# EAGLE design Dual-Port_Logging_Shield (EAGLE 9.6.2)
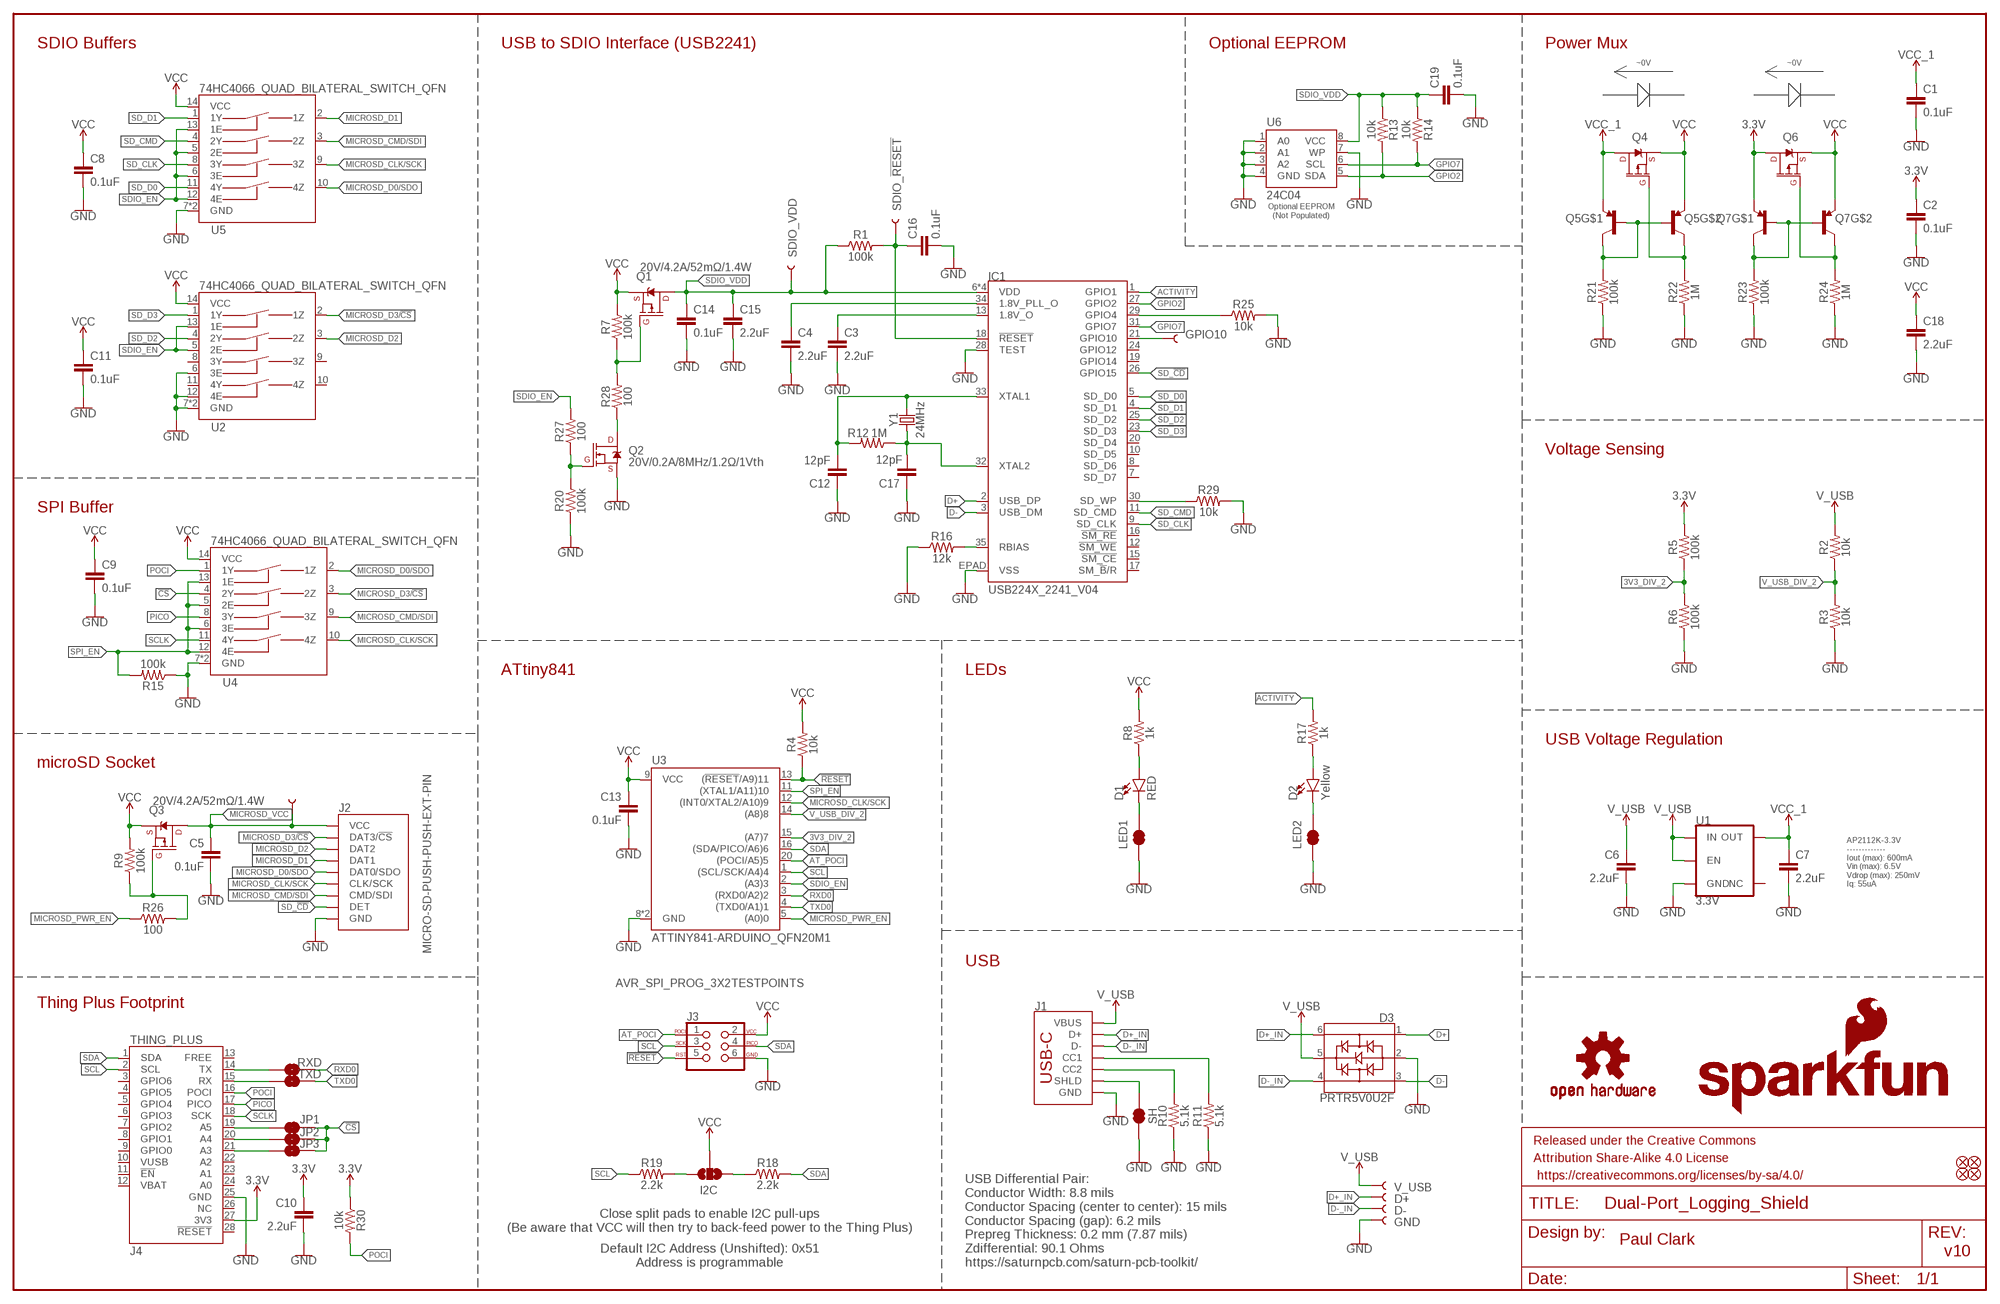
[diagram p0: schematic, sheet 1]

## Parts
C1  0.1uF  0.1UF-0402T-6.3V-10%-X7R  [0402-TIGHT]
C2  0.1uF  0.1UF-0402T-6.3V-10%-X7R  [0402-TIGHT]
C3  2.2uF  2.2UF-0402_TIGHT-10V-10%-X5R  [0402-TIGHT]
C4  2.2uF  2.2UF-0402_TIGHT-10V-10%-X5R  [0402-TIGHT]
C5  0.1uF  0.1UF-0402T-6.3V-10%-X7R  [0402-TIGHT]
C6  2.2uF  2.2UF-0402_TIGHT-10V-10%-X5R  [0402-TIGHT]
C7  2.2uF  2.2UF-0402_TIGHT-10V-10%-X5R  [0402-TIGHT]
C8  0.1uF  0.1UF-0402T-6.3V-10%-X7R  [0402-TIGHT]
C9  0.1uF  0.1UF-0402T-6.3V-10%-X7R  [0402-TIGHT]
C10  2.2uF  2.2UF-0402_TIGHT-10V-10%-X5R  [0402-TIGHT]
C11  0.1uF  0.1UF-0402T-6.3V-10%-X7R  [0402-TIGHT]
C12  12pF  12PF-0402T-50V-5%  [0402-TIGHT]
C13  0.1uF  0.1UF-0402T-6.3V-10%-X7R  [0402-TIGHT]
C14  0.1uF  0.1UF-0402T-6.3V-10%-X7R  [0402-TIGHT]
C15  2.2uF  2.2UF-0402_TIGHT-10V-10%-X5R  [0402-TIGHT]
C16  0.1uF  0.1UF-0402T-6.3V-10%-X7R  [0402-TIGHT]
C17  12pF  12PF-0402T-50V-5%  [0402-TIGHT]
C18  2.2uF  2.2UF-0402_TIGHT-10V-10%-X5R  [0402-TIGHT]
C19  0.1uF  0.1UF-0402T-6.3V-10%-X7R  [0402-TIGHT]
D1  RED  LED-RED0603  [LED-0603]
D2  Yellow  LED-YELLOW0603  [LED-0603]
D3  PRTR5V0U2F  [SOT886]
D+  TEST-POINT3X5  [PAD.03X.05]
D-  TEST-POINT3X5  [PAD.03X.05]
FD1  FIDUCIALUFIDUCIAL  [FIDUCIAL-MICRO]
FD2  FIDUCIALUFIDUCIAL  [FIDUCIAL-MICRO]
FD3  FIDUCIALUFIDUCIAL  [FIDUCIAL-MICRO]
FD4  FIDUCIALUFIDUCIAL  [FIDUCIAL-MICRO]
FRAME1  FRAME-LEDGER  [CREATIVE_COMMONS]
GND  TEST-POINT3X5  [PAD.03X.05]
GPIO10  TEST-POINT3  [PAD.03X.03]
I2C  JUMPER-SMT_3_NO_SILK  [SMT-JUMPER_3_NO_SILK]
IC1  USB224X_2241_V04  [36-QFN]
J1  USB_C_4-LAYER_PADS  [USB-C-16P_4LAYER-PADS]
J2  MICRO-SD-PUSH-PUSH-EXT-PIN  [MICROSD-EXTERNALPIN]
J3  AVR_SPI_PROG_3X2TESTPOINTS  [2X3_TEST_POINTS]
J4  THING_PLUS  [THING_PLUS]
JP1  JUMPER-SMT_2_NC_TRACE_SILK  [SMT-JUMPER_2_NC_TRACE_SILK]
JP2  JUMPER-SMT_2_NO_SILK  [SMT-JUMPER_2_NO_SILK]
JP3  JUMPER-SMT_2_NO_SILK  [SMT-JUMPER_2_NO_SILK]
LED1  JUMPER-SMT_2_NC_TRACE_SILK  [SMT-JUMPER_2_NC_TRACE_SILK]
LED2  JUMPER-SMT_2_NC_TRACE_SILK  [SMT-JUMPER_2_NC_TRACE_SILK]
LOGO2  OSHW-LOGOMINI  [OSHW-LOGO-MINI]
LOGO3  OSHW-LOGOMINI  [OSHW-LOGO-MINI]
LOGO4  SFE_LOGO_FLAME.2_INCH  [SFE_LOGO_FLAME_.2]
LOGO5  SFE_LOGO_NAME_FLAME.1_INCH  [SFE_LOGO_NAME_FLAME_.1]
MICROSD_VCC  TEST-POINT3  [PAD.03X.03]
Q1  20V/4.2A/52mΩ/1.4W  MOSFET_PCH-DMG2305UX-7  [SOT23-3]
Q2  20V/0.2A/8MHz/1.2Ω/1Vth  MOSFET-NCH-RE1C002UNTCL  [SOT-416FL]
Q3  20V/4.2A/52mΩ/1.4W  MOSFET_PCH-DMG2305UX-7  [SOT23-3]
Q4  20V/4.2A/52mΩ/1.4W  MOSFET_PCH-DMG2305UX-7  [SOT23-3]
Q5  TRANS_PNP_DUALSOT-363  [SOT363_PHILIPS]
Q6  20V/4.2A/52mΩ/1.4W  MOSFET_PCH-DMG2305UX-7  [SOT23-3]
Q7  TRANS_PNP_DUALSOT-363  [SOT363_PHILIPS]
R1  100k  100KOHM-0402T-1/16W-1%  [0402-TIGHT]
R2  10k  10KOHM-0402T-1/16W-1%  [0402-TIGHT]
R3  10k  10KOHM-0402T-1/16W-1%  [0402-TIGHT]
R4  10k  10KOHM-0402T-1/16W-1%  [0402-TIGHT]
R5  100k  100KOHM-0402T-1/16W-1%  [0402-TIGHT]
R6  100k  100KOHM-0402T-1/16W-1%  [0402-TIGHT]
R7  100k  100KOHM-0402T-1/16W-1%  [0402-TIGHT]
R8  1k  1KOHM-0402T-1/16W-1%  [0402-TIGHT]
R9  100k  100KOHM-0402T-1/16W-1%  [0402-TIGHT]
R10  5.1k  5.1KOHM-0402T-1/16W-1%  [0402-TIGHT]
R11  5.1k  5.1KOHM-0402T-1/16W-1%  [0402-TIGHT]
R12  1M  1MOHM-0402T-1/16W-5%  [0402-TIGHT]
R13  10k  10KOHM-0402T-1/16W-1%  [0402-TIGHT]
R14  10k  10KOHM-0402T-1/16W-1%  [0402-TIGHT]
R15  100k  100KOHM-0402T-1/16W-1%  [0402-TIGHT]
R16  12k  12KOHM-0603-1/10W-1%  [0603]
R17  1k  1KOHM-0402T-1/16W-1%  [0402-TIGHT]
R18  2.2k  2.2KOHM-0402T-1/16W-1%  [0402-TIGHT]
R19  2.2k  2.2KOHM-0402T-1/16W-1%  [0402-TIGHT]
R20  100k  100KOHM-0402T-1/16W-1%  [0402-TIGHT]
R21  100k  100KOHM-0402T-1/16W-1%  [0402-TIGHT]
R22  1M  1MOHM-0402T-1/16W-5%  [0402-TIGHT]
R23  100k  100KOHM-0402T-1/16W-1%  [0402-TIGHT]
R24  1M  1MOHM-0402T-1/16W-5%  [0402-TIGHT]
R25  10k  10KOHM-0402T-1/16W-1%  [0402-TIGHT]
R26  100  100OHM-0402-TIGHT-1/16W-1%  [0402-TIGHT]
R27  100  100OHM-0402-TIGHT-1/16W-1%  [0402-TIGHT]
R28  100  100OHM-0402-TIGHT-1/16W-1%  [0402-TIGHT]
R29  10k  10KOHM-0402T-1/16W-1%  [0402-TIGHT]
R30  10k  10KOHM-0402T-1/16W-1%  [0402-TIGHT]
RXD  JUMPER-SMT_2_NO_SILK  [SMT-JUMPER_2_NO_SILK]
SDIO_!RESET!  TEST-POINT3  [PAD.03X.03]
SDIO_VDD  TEST-POINT3  [PAD.03X.03]
SH  JUMPER-SMT_2_NC_TRACE_SILK  [SMT-JUMPER_2_NC_TRACE_SILK]
TXD  JUMPER-SMT_2_NO_SILK  [SMT-JUMPER_2_NO_SILK]
U1  3.3V  V_REG_AP2112K-3.3V  [SOT23-5]
U2  74HC4066_QUAD_BILATERAL_SWITCH_QFN  [14-QFN]
U3  ATTINY841-ARDUINO_QFN20M1  [QFN20_20M1]
U4  74HC4066_QUAD_BILATERAL_SWITCH_QFN  [14-QFN]
U5  74HC4066_QUAD_BILATERAL_SWITCH_QFN  [14-QFN]
U6  24C04  EEPROM-I2C256K  [SO08]
V_USB  TEST-POINT3X5  [PAD.03X.05]
Y1  24MHz  CRYSTAL-24MHZ-SMD-2.0X1.6MM  [CRYSTAL-SMD-2.0X1.6MM]

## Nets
3.3V: C2.1 C10.1 J4.27(3V3) Q6.3(D) Q7.1(E) R5.2 R30.1
3V3_DIV_2: R5.1 R6.2 U3.15((A7)7)
!CS!: JP1.2 JP2.2 JP3.2 U4.4(2Y)
!RESET!: J3.5 R4.1 U3.13((!RESET!/A9)11)
ACTIVITY: IC1.1(GPIO1) R17.2
AT_POCI: J3.1 U3.20((POCI/A5)5)
D+: D3.1 IC1.2(USB_DP)
D+_IN: D3.6 D+.1 J1.A6(D+) J1.B6(D+)
D-: D3.3 IC1.3(USB_DM)
D-_IN: D3.4 D-.1 J1.A7(D-) J1.B7(D-)
GND: C1.2 C2.2 C3.2 C4.2 C5.2 C6.2 C7.2 C8.2 C9.2 C10.2 C11.2 C12.1 C13.2 C14.2 C15.2 C16.2 C17.1 C18.2 C19.2 D3.2 GND.1 IC1.28(TEST) IC1.EPAD(VSS) J1.GND J1.GND2(GND) J2.6(GND) J2.10(GND) J2.11(GND) J2.12(GND) J2.13(GND) J3.6 J4.25(GND) LED1.1 LED2.1 Q2.2(S) R3.1 R6.1 R10.1 R11.1 R15.1 R16.1 R20.1 R21.1 R22.1 R23.1 R24.1 R25.2 R29.2 SH.2 U1.2(GND) U2.6(3E) U2.7(GND) U2.12(4E) U2.EPAD(GND) U3.8(GND) U3.PAD(GND) U4.7(GND) U4.EPAD(GND) U5.7(GND) U5.EPAD(GND) U6.1(A0) U6.2(A1) U6.3(A2) U6.4(GND) U6.7(WP)
GPIO2: IC1.27(GPIO2) R13.2 U6.5(SDA)
GPIO4: IC1.29(GPIO4) R25.1
GPIO7: IC1.31(GPIO7) R14.2 U6.6(SCL)
GPIO10: GPIO10.1 IC1.21(GPIO10)
MICROSD_CLK/SCK: J2.5(CLK/SCK) U3.12((INT0/XTAL2/A10)9) U4.10(4Z) U5.9(3Z)
MICROSD_CMD/SDI: J2.3(CMD/SDI) U4.9(3Z) U5.3(2Z)
MICROSD_D0/SDO: J2.7(DAT0/SDO) U4.2(1Z) U5.10(4Z)
MICROSD_D1: J2.8(DAT1) U5.2(1Z)
MICROSD_D2: J2.1(DAT2) U2.3(2Z)
MICROSD_D3/!CS!: J2.2(DAT3/!CS!) U2.2(1Z) U4.3(2Z)
MICROSD_PWR_EN: R26.1 U3.5((A0)0)
MICROSD_VCC: C5.1 J2.4(VCC) MICROSD_VCC.1 Q3.3(D)
N$1: J1.A5(CC1) R11.2
N$2: J1.B5(CC2) R10.2
N$3: C3.1 IC1.13(1.8V_O)
N$4: C4.1 IC1.34(1.8V_PLL_O)
N$5: Q5.2(B) Q5.5(B) Q5.6(C) R21.2
N$6: Q3.1(G) R9.1 R26.2
N$7: Q2.1(G) R20.2 R27.1
N$8: Q2.3(D) R28.1
N$9: J4.19(A5) JP1.1
N$10: J4.20(A4) JP2.1
N$11: J4.21(A3) JP3.1
N$12: J1.SHLD1(SHLD) J1.SHLD2(SHLD) J1.SHLD3(SHLD) J1.SHLD4(SHLD) SH.1
N$13: Q4.1(G) Q5.3(C) R22.2
N$14: I2C.3 R19.2
N$15: Q7.2(B) Q7.5(B) Q7.6(C) R23.2
N$16: I2C.1 R18.1
N$17: Q1.1(G) R7.1 R28.2
N$18: D2.A R17.1
N$19: D2.C LED2.2
N$20: IC1.30(SD_WP) R29.1
N$22: D1.A R8.1
N$23: IC1.35(RBIAS) R16.2
N$25: J4.14(TX) RXD.1
N$26: J4.15(RX) TXD.1
N$27: D1.C LED1.2
N$28: Q6.1(G) Q7.3(C) R24.2
PICO: J4.17(PICO) U4.8(3Y)
POCI: J4.16(POCI) R30.2 U4.1(1Y)
RXD0: RXD.2 U3.3((RXD0/A2)2)
SCL: J3.3 J4.2(SCL) R19.1 U3.1((SCL/SCK/A4)4)
SCLK: J4.18(SCK) U4.11(4Y)
SD_!CD!: IC1.26(GPIO15) J2.9(DET)
SD_CLK: IC1.9(SD_CLK) U5.8(3Y)
SD_CMD: IC1.11(SD_CMD) U5.4(2Y)
SD_D0: IC1.5(SD_D0) U5.11(4Y)
SD_D1: IC1.4(SD_D1) U5.1(1Y)
SD_D2: IC1.25(SD_D2) U2.4(2Y)
SD_D3: IC1.23(SD_D3) U2.1(1Y)
SDA: J3.4 J4.1(SDA) R18.2 U3.16((SDA/PICO/A6)6)
SDIO_!RESET!: C16.1 IC1.18(!RESET!) R1.2 SDIO_!RESET!.1
SDIO_EN: R27.2 U2.5(2E) U2.13(1E) U3.2((A3)3) U5.5(2E) U5.6(3E) U5.12(4E) U5.13(1E)
SDIO_VDD: C14.1 C15.1 C19.1 IC1.6(VDD) IC1.14(VDD) IC1.22(VDD) IC1.36(VDD) Q1.3(D) R1.1 R13.1 R14.1 SDIO_VDD.1 U6.8(VCC)
SPI_EN: R15.2 U3.11((XTAL1/A11)10) U4.5(2E) U4.6(3E) U4.12(4E) U4.13(1E)
TXD0: TXD.2 U3.4((TXD0/A1)1)
V_USB: C6.1 D3.5 J1.VBUS1(VBUS) J1.VBUS2(VBUS) R2.2 U1.1(IN) U1.3(EN) V_USB.1
V_USB_DIV_2: R2.1 R3.2 U3.14((A8)8)
VCC: C8.1 C9.1 C11.1 C13.1 C18.1 I2C.2 J3.2 Q1.2(S) Q3.2(S) Q4.2(S) Q5.4(E) Q6.2(S) Q7.4(E) R4.2 R7.2 R8.2 R9.2 U2.14(VCC) U3.9(VCC) U4.14(VCC) U5.14(VCC)
VCC_1: C1.1 C7.1 Q4.3(D) Q5.1(E) U1.5(OUT)
XTAL1: C12.2 IC1.33(XTAL1) R12.2 Y1.3
XTAL2: C17.2 IC1.32(XTAL2) R12.1 Y1.1
Unconnected: IC1.7(SD_D7) IC1.8(SD_D6) IC1.10(SD_D5) IC1.12(!SM_WE!) IC1.15(!SM_CE!) IC1.16(!SM_RE!) IC1.17(SM_!B!/R) IC1.19(GPIO14) IC1.20(SD_D4) IC1.24(GPIO12) J4.3(GPIO6) J4.4(GPIO5) J4.5(GPIO4) J4.6(GPIO3) J4.7(GPIO2) J4.8(GPIO1) J4.9(GPIO0) J4.10(VUSB) J4.11(!EN) J4.12(VBAT) J4.13(FREE) J4.22(A2) J4.23(A1) J4.24(A0) J4.26(NC) J4.28(!RESET) U1.4(NC) U2.8(3Y) U2.9(3Z) U2.10(4Z) U2.11(4Y)

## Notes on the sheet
- SDIO Buffers | USB to SDIO Interface (USB2241) | Optional EEPROM | Power Mux
- ~0V | ~0V
- Optional EEPROM
  (Not Populated)
- Voltage Sensing
- SPI Buffer
- ATtiny841 | LEDs
- USB Voltage Regulation
- microSD Socket
- AP2112K-3.3V
  -------------
  Iout (max): 600mA 
  Vin (max): 6.5V
  Vdrop (max): 250mV
  Iq: 55uA
- USB
- Thing Plus Footprint
- USB Differential Pair:
  Conductor Width: 8.8 mils
  Conductor Spacing (center to center): 15 mils
  Conductor Spacing (gap): 6.2 mils
  Prepreg Thickness: 0.2 mm (7.87 mils)
  Zdifferential: 90.1 Ohms
  https://saturnpcb.com/saturn-pcb-toolkit/
- Close split pads to enable I2C pull-ups
  (Be aware that VCC will then try to back-feed power to the Thing Plus)
- Paul Clark
- v10
- Default I2C Address (Unshifted): 0x51
  Address is programmable

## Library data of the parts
C1 C2 C5 C8 C9 C11 C13 C14 C16 C19 = SparkFun-Capacitors:0.1UF: 0.1µF ceramic capacitors; PROD_ID: CAP-14993
C3 C4 C6 C7 C10 C15 C18 = SparkFun-Capacitors:2.2UF: 2.2µF ceramic capacitors; PROD_ID: CAP-14232
C12 C17 = SparkFun-Capacitors:12PF: 12pF ceramic capacitors; PROD_ID: CAP-14665
D1 = SparkFun-LED:LED-RED: Red SMD LED; PROD_ID: DIO-00819
D2 = SparkFun-LED:LED-YELLOW: Yellow SMD LED; PROD_ID: DIO-09003
D3 = SparkFun-IC-Power:PRTR5V0U2: A small ESD protection device. Most commonly used on USB D+/D- signals to protect large, expensive, or especially sensitive USB enabled devices.; PROD_ID: DIO-14084
D+ D- GND GPIO10 MICROSD_VCC SDIO_!RESET! SDIO_VDD V_USB = SparkFun-Connectors:TEST-POINT: SparkFun Test Points
FD1-FD4 = SparkFun-Aesthetics:FIDUCIAL: Fiducial Alignment Points
FRAME1 = SparkFun-Aesthetics:FRAME-LEDGER: Schematic Frame - Ledger
I2C = SparkFun-Jumpers:JUMPER-SMT_3_NO: Normally open jumper This jumper has three pads in close proximity to each other. Apply solder to close the connection(s).
IC1 = SparkFun-IC-Special-Function:USB224X: Microchip Technology USB224x Flash Media Controller 36-QFN Source: Datasheet; PROD_ID: IC-16527
J1 = SparkFun-Connectors:USB_C: USB Type C 16Pin Connector Super Speed pins not available on the 16-pin purely SMD connector so this part is best for USB 2.0 implementations. D1 and D2 are tied together enabling D+/- no matter which way the cable is plugged into the connector. The two channel configuration pins (CC1/2) are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; PROD_ID: CONN-14122
J2 = SparkFun-Connectors:MICRO-SD: microSD Socket for Transflash Various sockets for µSD. tDoc lines correctly indicate media card edge positions when inserting (unlocked, locked, depressed). NOTE: CD1 and CD2 are connected internally, and the default detect state of the socket is detect pin to ground. SparkFun Products: WAV Trigger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; PROD_ID: CONN-16110
J3 = SparkFun-Connectors:AVR_SPI_PROG_3X2: AVR ISP 6 Pin This is the reduced ISP connector for AVR programming. Common on Arduino. This footprint will take up less PCB space and can be used with a 10-pin to 6-pin adapter such as SKU: BOB-08508 **Special note about "TEST_POINT" package. The stop mask is on the top side, so if you want your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
J4 = Thing_Plus:THING_PLUS
JP1 LED1 LED2 SH = SparkFun-Jumpers:JUMPER-SMT_2_NC_TRACE: Normally closed trace jumper
JP2 JP3 RXD TXD = SparkFun-Jumpers:JUMPER-SMT_2_NO: Normally open jumper
LOGO2 LOGO3 = SparkFun-Aesthetics:OSHW-LOGO: Open-Source Hardware (OSHW) Logo
LOGO4 = SparkFun-Aesthetics:SFE_LOGO_FLAME: SparkFun Flame Logo
LOGO5 = SparkFun-Aesthetics:SFE_LOGO_NAME_FLAME: SparkFun Font Logo w/ Flame
Q1 Q3 Q4 Q6 = SparkFun-DiscreteSemi:MOSFET_PCH: P-channel MOSFETs Voltage controlled devices that allow control of high current outputs. SparkFun Products: SparkFun ESP32 Thing SparkFun ESP8266 Thing SparkFun Pi Servo HAT V2 DMG2305UX-7 (20V/4.2A/SOT23-3); PROD_ID: TRANS-14388
Q2 = SparkFun-DiscreteSemi:MOSFET-NCH: N-channel MOSFETs Voltage controlled devices that allow control of high current outputs. SparkFun Products: SparkFun OpenScale SparkFun Digital Sandbox SparkFun Monster Moto Shield SparkFun MOSFET Power Controller; PROD_ID: TRANS-14399
Q5 Q7 = SparkFun-DiscreteSemi:TRANS_PNP_DUAL: Dual PNP Transistors in Single Package The BCM857BS puts two PNP transistors in a single package. Bipolar (BJT) Transistor Array 2 PNP (Dual) 45V 100mA 100MHz 200mW Surface Mount SOT-363 Datasheet SparkFun Products: SparkFun Pi Servo HAT V2; PROD_ID: TRANS-14386
R1 R5-R7 R9 R15 R20 R21 R23 = SparkFun-Resistors:100KOHM: 100kΩ resistor; PROD_ID: RES-13495
R2-R4 R13 R14 R25 R29 R30 = SparkFun-Resistors:10KOHM: 10kΩ resistor; PROD_ID: RES-14241
R8 R17 = SparkFun-Resistors:1KOHM: 1kΩ resistor; PROD_ID: RES-14342
R10 R11 = SparkFun-Resistors:5.1KOHM; PROD_ID: RES-14340
R12 R22 R24 = SparkFun-Resistors:1MOHM: 1MΩ resistor; PROD_ID: RES-15185
R16 = SparkFun-Resistors:12KOHM: 12kΩ resistor; PROD_ID: RES-10327
R18 R19 = SparkFun-Resistors:2.2KOHM: 2.2kΩ resistor; PROD_ID: RES-14341
R26-R28 = SparkFun-Resistors:100OHM: 100Ω resistor; PROD_ID: RES-14962
U1 = SparkFun-IC-Power:V_REG_AP2112: AP2112 - 600mA CMOS LDO Regulator w/ Enable The AP2112 is CMOS process low dropout linear regulator with enable function, the regulator delivers a guaranteed 600mA (min.) continuous load current. Features Output Voltage Accuracy: ±1.5% Output Current: 600mA (Min.) Foldback Short Current Protection: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; PROD_ID: VREG-12457
U2 U4 U5 = SparkFun-IC-Logic:74HC4066_QUAD_BILATERAL_SWITCH: Nexperia Quad Bilateral Switch The 74HC4066 is a quad single pole, single throw analog switch. Each switch features two input/output terminals (nY and nZ) and an active HIGH enable input (nE). When nE is LOW, the analog switch is turned off. Inputs include clamp diodes. This enables the use of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; PROD_ID: IC-16528
U3 = SparkFun-IC-Microcontroller:ATTINY841-ARDUINO: ATtiny841; DIGIKEY_PART: ATTINY841-MU-ND; PROD_ID: IC-16067
U6 = SparkFun-IC-Memory:EEPROM-I2C: I2C EEPROMs, 24LC256 and others 24LC256 Series 256 kb I2C 2 Wire (32 k x 8 Bit) 2.5 V Serial EEPROM SMD - SOIC-8 Datasheet SparkFun Products SparkFun UDB5 - PIC UAV Development Board (GPS-11703); PROD_ID: IC-09714; VALUE: 24LC256
Y1 = SparkFun-Clocks:CRYSTAL-24MHZ: 24MHz Crystal; PROD_ID: XTAL-14845

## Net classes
1 Power: width 0.305 mm
2 3.3V: width 0.508 mm

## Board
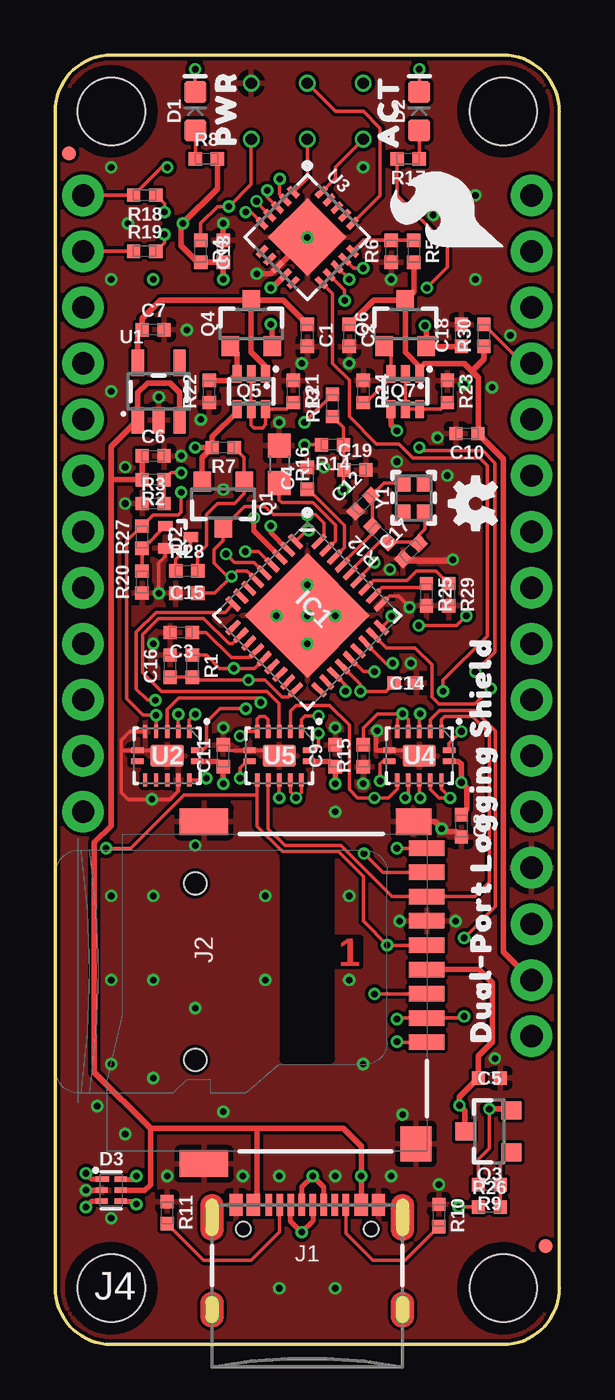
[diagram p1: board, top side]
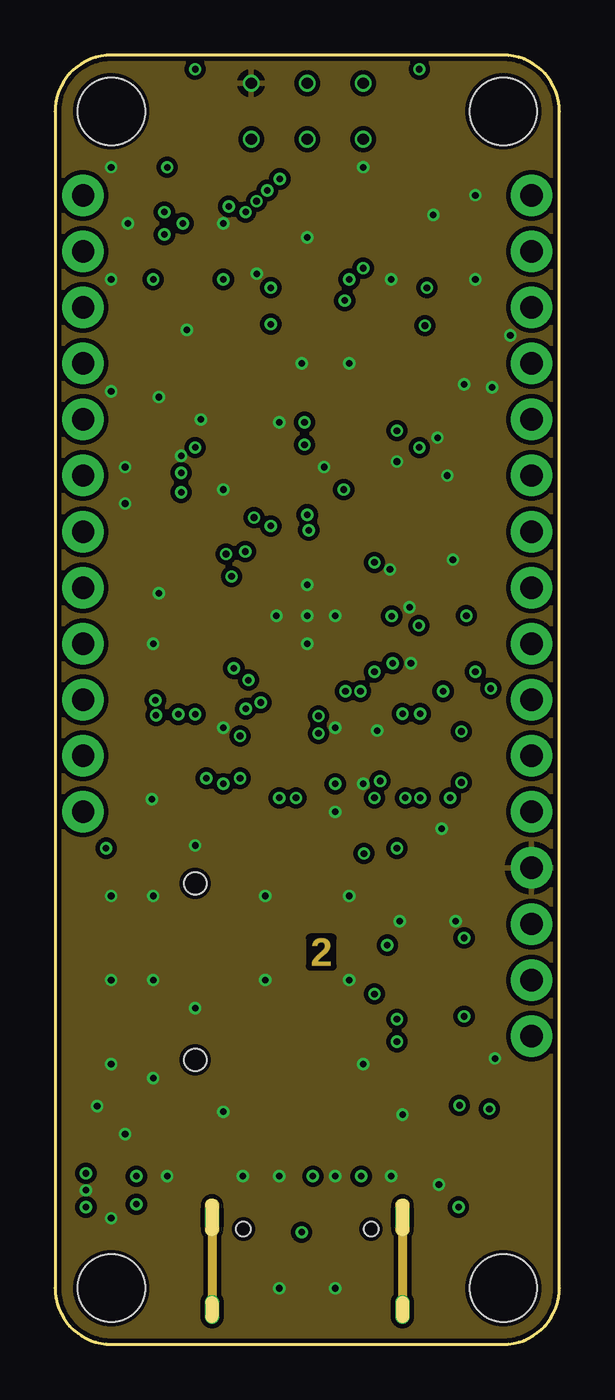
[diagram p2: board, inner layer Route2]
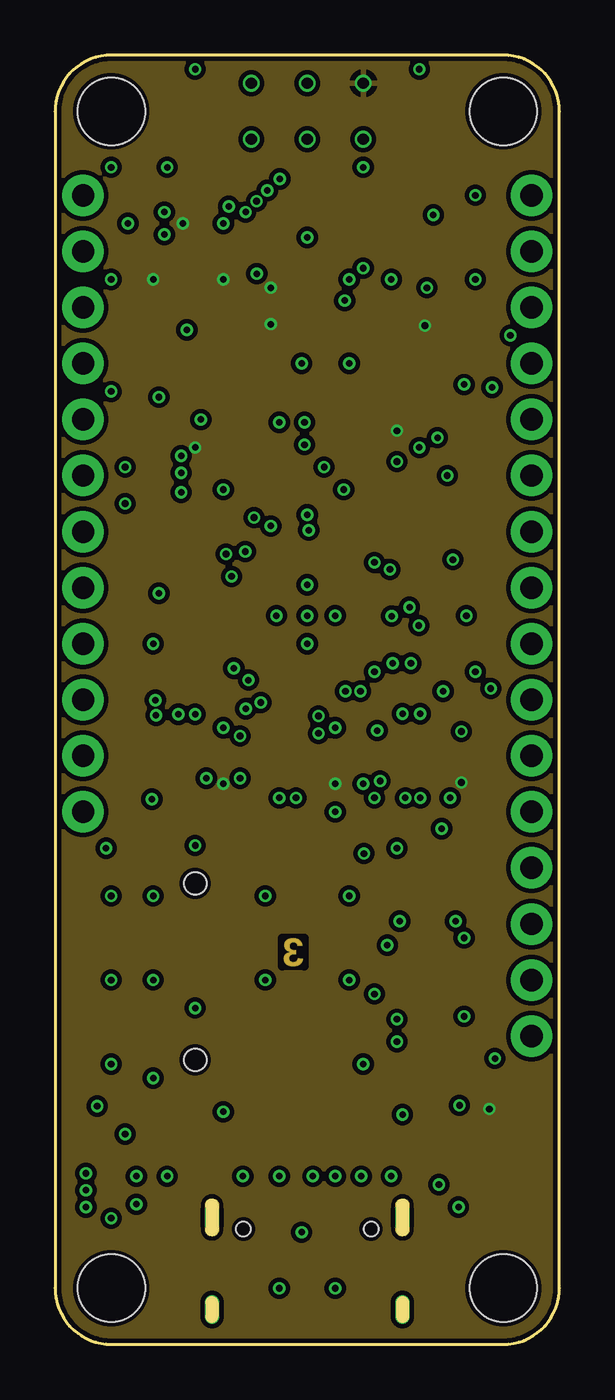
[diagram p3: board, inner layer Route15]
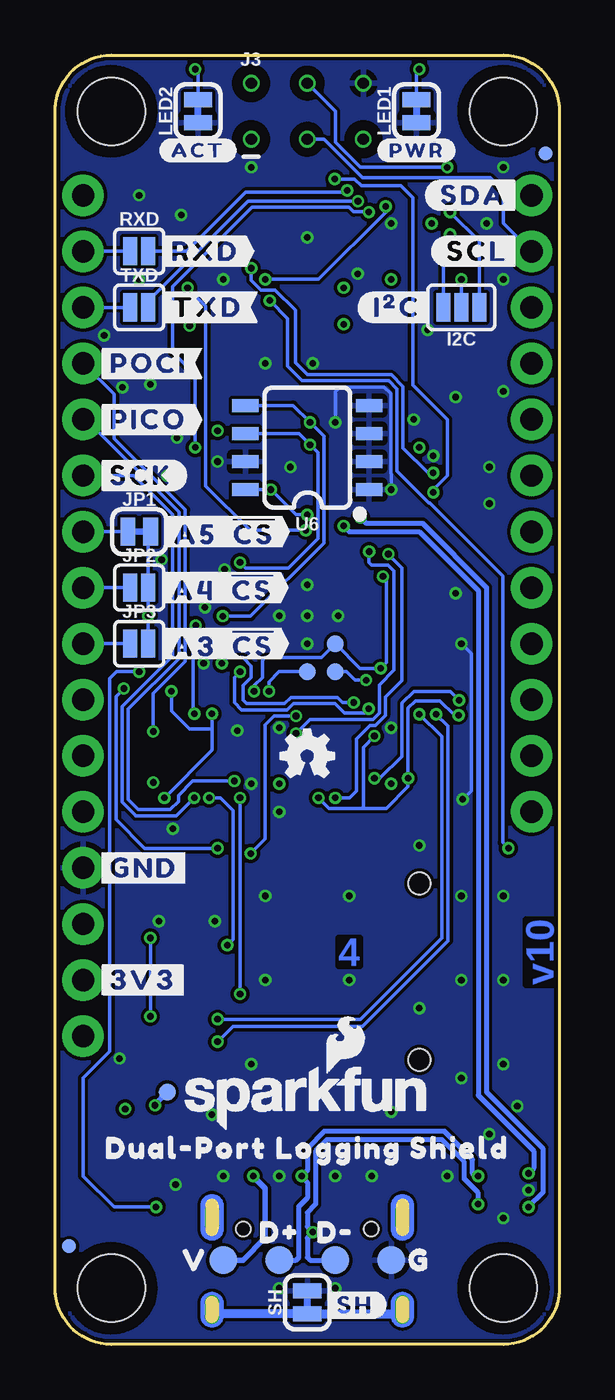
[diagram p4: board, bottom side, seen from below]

Size 22.86 x 58.42 mm. Coordinates in mm from the lower left corner, seen from the top.
Outline: 0,2.54 arc90 2.54,0 20.32,0 arc90 22.86,2.54 22.86,55.88 arc90 20.32,58.42 2.54,58.42 arc90 0,55.88 0,2.54
Copper layers (1*2*15*16): Top 0.035559375mm / dielectric 0.47751875mm / Route2 0.035559375mm / dielectric 0.47751875mm / Route15 0.035559375mm / dielectric 0.47751875mm / Bottom 0.035559375mm
Design rules "SparkFun-4-Layer-Minimum-JLCPCB": minimum track width 5mil, minimum drill 0.2mm, track to track 5mil, track to pad 5mil, pad to pad 5mil, via to via 5mil, smd to smd 5mil, copper to edge 7mil, drill to drill 7mil, minimum pad ring 5mil, minimum via ring 5mil, stop-mask expansion 2.5mil, vias tented up to drill 25mil, thermal gap 10mil
tRestrict: area 10.4,13 to 12.4,22
bRestrict: area 8.3,54 to 9.5,55.2; area 13.3,54 to 14.6,55.2; area 13.3,56.5 to 14.6,57.8; 2 lines

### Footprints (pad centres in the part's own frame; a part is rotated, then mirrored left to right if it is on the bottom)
0402-TIGHT = smd 0.6 x 0.6: 1 -0.5,0; 2 0.5,0
LED-0603 = smd 1 x 1: A -0.877,0; C 0.877,0
SOT886 = smd 0.61 x 0.25: 1 -0.405,0.5 | smd 0.56 x 0.25: 2 -0.43,0; 3 -0.43,-0.5; 4 0.43,-0.5; 5 0.43,0; 6 0.43,0.5
PAD.03X.05 = smd 1.27 x 1.27: 1 0,0
FIDUCIAL-MICRO = smd 0.635 x 0.635: 1 0,0
PAD.03X.03 = smd 0.762 x 0.762: 1 0,0
SMT-JUMPER_3_NO_SILK = smd 0.635 x 1.27: 1 -0.813,0; 2 0,0; 3 0.813,0
36-QFN = smd 0.8 x 0.25: 1 -2.75,2; 2 -2.75,1.5; 3 -2.75,1; 4 -2.75,0.5; 5 -2.75,0; 6 -2.75,-0.5; 7 -2.75,-1; 8 -2.75,-1.5; 9 -2.75,-2; 19 2.75,-2; 20 2.75,-1.5; 21 2.75,-1; 22 2.75,-0.5; 23 2.75,0; 24 2.75,0.5; 25 2.75,1; 26 2.75,1.5; 27 2.75,2 | smd 0.25 x 0.8: 10 -2,-2.75; 11 -1.5,-2.75; 12 -1,-2.75; 13 -0.5,-2.75; 14 0,-2.75; 15 0.5,-2.75; 16 1,-2.75; 17 1.5,-2.75; 18 2,-2.75; 28 2,2.75; 29 1.5,2.75; 30 1,2.75; 31 0.5,2.75; 32 0,2.75; 33 -0.5,2.75; 34 -1,2.75; 35 -1.5,2.75; 36 -2,2.75 | smd 4 x 4: EPAD 0,0
USB-C-16P_4LAYER-PADS = smd 0.3 x 1: A5 -1.25,-0.34; A6 -0.25,-0.34; A7 0.25,-0.34; A8 1.25,-0.34; B5 1.75,-0.34; B6 0.75,-0.34; B7 -0.75,-0.34; B8 -1.75,-0.34 | smd 0.6 x 1: GND -3.225,-0.34; GND2 3.225,-0.34; VBUS1 -2.45,-0.34; VBUS2 2.45,-0.34 | drill 0.4 pad 0.6 long: SHLD1 -4.318,-0.915; SHLD2 4.318,-0.915; SHLD3 -4.318,-5.095; SHLD4 4.318,-5.095 | hole 0.65: -2.89,-1.445; 2.89,-1.445
MICROSD-EXTERNALPIN = smd 0.7 x 1.6: 1 2.25,10.5; 2 1.15,10.5; 3 0.05,10.5; 4 -1.05,10.5; 5 -2.15,10.5; 6 -3.25,10.5; 7 -4.35,10.5; 8 -5.45,10.5; 9 -6.55,10.5 | smd 1.2 x 1.6: 10 -7.75,9.9 | smd 1.2 x 2.2: 11 -7.75,0.4; 12 7.75,0.4 | smd 1.6 x 1.4: 13 6.85,10 | hole 1: 3.05,0; -4.95,0
2X3_TEST_POINTS = drill 0.508: 1 -2.54,-1.27; 2 -2.54,1.27; 3 0,-1.27; 4 0,1.27; 5 2.54,-1.27; 6 2.54,1.27
THING_PLUS = drill 1.016 pad 1.88: 1 1.27,52.07; 2 1.27,49.53; 3 1.27,46.99; 4 1.27,44.45; 5 1.27,41.91; 6 1.27,39.37; 7 1.27,36.83; 8 1.27,34.29; 9 1.27,31.75; 10 1.27,29.21; 11 1.27,26.67; 12 1.27,24.13; 13 21.59,52.07; 14 21.59,49.53; 15 21.59,46.99; 16 21.59,44.45; 17 21.59,41.91; 18 21.59,39.37; 19 21.59,36.83; 20 21.59,34.29; 21 21.59,31.75; 22 21.59,29.21; 23 21.59,26.67; 24 21.59,24.13; 25 21.59,21.59; 26 21.59,19.05; 27 21.59,16.51; 28 21.59,13.97 | hole 3.048: 2.54,2.54; 2.54,55.88; 20.32,2.54; 20.32,55.88
SMT-JUMPER_2_NC_TRACE_SILK = smd 0.66 x 1.27: 1 -0.521,0; 2 0.521,0
SMT-JUMPER_2_NO_SILK = smd 0.635 x 1.27: 1 -0.406,0; 2 0.406,0
SOT23-3 = smd 0.8 x 0.9: 1 -0.95,-1; 2 0.95,-1; 3 0,1.1
SOT-416FL = smd 0.46 x 0.65: 1 -0.5,-1.1; 2 0.5,-1.1; 3 0,0.05
SOT363_PHILIPS = smd 0.4 x 0.8: 1 -0.65,-0.8; 2 0,-0.8; 3 0.65,-0.8; 4 0.65,0.8; 5 0,0.8; 6 -0.65,0.8
0603 = smd 1.1 x 1: 1 -0.85,0; 2 0.85,0
SOT23-5 = smd 0.55 x 1.2: 1 -0.95,-1.3; 2 0,-1.3; 3 0.95,-1.3; 4 0.95,1.3; 5 -0.95,1.3
14-QFN = smd 0.25 x 0.6: 1 -0.25,1.35; 7 -0.25,-1.35; 8 0.25,-1.35; 14 0.25,1.35 | smd 0.6 x 0.25: 2 -1.1,1; 3 -1.1,0.5; 4 -1.1,0; 5 -1.1,-0.5; 6 -1.1,-1; 9 1.1,-1; 10 1.1,-0.5; 11 1.1,0; 12 1.1,0.5; 13 1.1,1 | smd 1 x 1.5: EPAD 0,0
QFN20_20M1 = smd 0.6 x 0.25: 1 -1.9,1; 2 -1.9,0.5; 3 -1.9,0; 4 -1.9,-0.5; 5 -1.9,-1; 11 1.9,-1; 12 1.9,-0.5; 13 1.9,0; 14 1.9,0.5; 15 1.9,1 | smd 0.25 x 0.6: 6 -1,-1.9; 7 -0.5,-1.9; 8 0,-1.9; 9 0.5,-1.9; 10 1,-1.9; 16 1,1.9; 17 0.5,1.9; 18 0,1.9; 19 -0.5,1.9; 20 -1,1.9 | smd 2.5 x 2.5: PAD 0,0
SO08 = smd 0.6 x 1.2: 1 -1.905,-2.8; 2 -0.635,-2.8; 3 0.635,-2.8; 4 1.905,-2.8; 5 1.905,2.8; 6 0.635,2.8; 7 -0.635,2.8; 8 -1.905,2.8
CRYSTAL-SMD-2.0X1.6MM = smd 0.75 x 0.7: 1 -0.675,-0.5; 2 0.675,-0.5; 3 0.675,0.5; 4 -0.675,0.5

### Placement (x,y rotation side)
C1  11.43,45.72 270 top
C2  13.34,45.72 270 top
C3  5.71,32.26 180 top
C4  11.43,39.24 90 top
C5  19.68,12.06 0 top
C6  4.45,40.26 0 top
C7  4.45,45.97 0 top
C8  18.41,23.5 270 top
C9  12.7,26.67 90 top
C10  18.67,41.27 180 top
C11  7.62,26.67 90 top
C12  13.97,38.1 45 top
C13  7.62,49.53 90 top
C14  15.88,29.97 0 top
C15  5.97,34.04 180 top
C16  5.21,30.73 90 top
C17  16.13,35.94 45 top
C18  18.41,45.72 90 top
C19  13.59,39.62 0 top
D1  6.35,55.88 90 top
D2  16.51,55.88 90 top
D3  2.54,6.99 0 top
D+  12.7,3.81 0 bottom
D-  10.16,3.81 0 bottom
FD1  0.64,53.98 0 top
FD2  22.23,4.45 0 bottom
FD3  22.23,4.45 0 top
FD4  0.64,53.98 0 bottom
FRAME1  not placed on the board
GND  7.62,3.81 0 bottom
GPIO10  11.43,30.48 0 bottom
I2C  4.45,46.99 180 bottom
IC1  11.43,33.02 315 top
J1  11.43,6.67 0 top
J2  6.35,15.94 270 top
J3  11.43,55.88 0 bottom
J4  0,0 0 top
JP1  19.05,36.83 0 bottom
JP2  19.05,34.29 0 bottom
JP3  19.05,31.75 0 bottom
LED1  6.48,55.88 90 bottom
LED2  16.38,55.88 90 bottom
LOGO1  SPECIAL_INSTRUCTIONS-ORDERING  [ORDERING_INSTRUCTIONS]  not placed on the board
LOGO2  19.05,38.1 90 top
LOGO3  11.43,26.67 0 bottom
LOGO4  17.78,51.44 90 top
LOGO5  11.43,11.18 0 bottom
MICROSD_VCC  17.78,11.43 0 bottom
Q1  7.62,38.1 180 top
Q2  6.1,36.58 270 top
Q3  19.68,9.65 90 top
Q4  8.89,46.23 0 top
Q5  8.89,43.18 180 top
Q6  15.88,46.23 0 top
Q7  15.88,43.18 180 top
R1  6.22,30.73 270 top
R2  4.45,39.18 180 top
R3  4.45,38.1 0 top
R4  6.6,49.53 270 top
R5  16.26,49.53 270 top
R6  15.24,49.53 90 top
R7  7.62,40.64 180 top
R8  6.86,53.72 0 top
R9  19.68,7.24 180 top
R10  17.4,5.84 270 top
R11  5.08,5.97 270 top
R12  14.73,36.7 135 top
R13  12.57,42.55 90 top
R14  12.57,40.77 180 top
R15  13.97,26.67 90 top
R16  10.16,39.88 270 top
R17  16,53.72 180 top
R18  4.06,52.07 180 top
R19  4.06,49.53 0 top
R20  3.94,34.54 90 top
R21  10.79,43.18 270 top
R22  6.99,43.18 90 top
R23  17.78,43.18 270 top
R24  13.97,43.18 270 top
R25  16.83,33.97 270 top
R26  19.68,6.22 0 top
R27  3.94,36.58 90 top
R28  5.97,35.05 0 top
R29  17.84,33.97 270 top
R30  19.43,45.72 90 top
RXD  19.05,49.53 0 bottom
SDIO_!RESET!  10.16,30.48 0 bottom
SDIO_VDD  10.16,31.75 0 bottom
SH  11.43,1.91 90 bottom
TXD  19.05,46.99 0 bottom
U1  4.7,43.18 0 top
U2  5.08,26.67 270 top
U3  11.43,50.16 315 top
U4  16.51,26.67 270 top
U5  10.16,26.67 270 top
U6  11.43,40.64 90 bottom
U$1  [#SDA#0]  1.65,52.07 0 bottom
U$2  [#SCL#1]  1.65,49.53 0 bottom
U$3  [#POCI#0]  21.08,44.45 0 bottom
U$4  [#PICO#1]  21.08,41.91 0 bottom
U$5  [#SCK#2]  21.08,39.37 0 bottom
U$6  [DUAL#PORT_LOGGING_SHIELD0]  11.43,8.89 0 bottom
U$7  [#GND#0]  21.08,21.59 0 bottom
U$8  [#3V3#1]  21.08,16.51 0 bottom
U$9  [#RXD#0]  18.29,49.53 0 bottom
U$10  [#TXD#1]  18.29,46.99 0 bottom
U$11  [PWR0]  7.75,56.01 90 top
U$12  [ACT0]  15.11,55.88 90 top
U$13  [#I�C#0]  7.37,46.99 0 bottom
U$14  [DUAL#PORT_LOGGING_SHIELD0]  19.3,22.86 90 top
U$15  [#PWR#0]  6.48,54.1 0 bottom
U$16  [#ACT#0]  16.38,54.1 0 bottom
U$17  [#A5__#CS##0]  18.16,36.83 0 bottom
U$18  [#A4__#CS##6]  18.29,34.29 0 bottom
U$19  [#A3__#CS##6]  18.29,31.75 0 bottom
U$20  [#SH#0]  9.27,1.78 0 bottom
U$21  [G0]  6.35,3.81 0 bottom
U$22  [V0]  16.51,3.81 0 bottom
U$23  [D#0]  10.16,5.08 0 bottom
U$25  [D#1]  12.7,5.08 0 bottom
V_USB  15.24,3.81 0 bottom
Y1  16.26,38.35 90 top

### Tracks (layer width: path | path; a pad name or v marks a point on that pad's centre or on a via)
3.3V
  Top 0.254: J4.27 20.32,17.78 20.32,40.12 C10.1 19.18,41.28 19.18,43.81 18.89,44.1 | 18.89,44.1 18.54,44.45 16.74,44.45 16.52,44.23 Q7.1 16.52,44.31 15.88,44.96 Q6.3 | C2.1 14.44,47.33 Q6.3 | R5.2 16.26,47.71 Q6.3 | R30.1 19.43,44.64 18.89,44.1
3V3_DIV_2
  Top 0.152: R5.1 R6.2 13.98,50.03 U3.15
!CS!  (via drill 0.3)
  Top 0.152: v16.49,32.58 18.2,32.58 v18.64,33.02 | U4.4 16.51,28.54 v16.55,28.58
  Bottom 0.152: JP3.2 v18.64,33.02 JP2.2 18.64,36.72 JP1.2 | v16.55,28.58 16.61,28.64 16.61,32.45 v16.49,32.58
!RESET!  (via drill 0.3)
  Top 0.152: U3.13 v13.34,48.26 | v13.34,48.26 | J3.5 8.89,52.58 v7.87,51.56 7.37,51.56 6.6,50.8 R4.1
  Bottom 0.152: v13.34,48.26 10.92,48.26 7.87,51.31 v7.87,51.56
ACTIVITY  (via drill 0.3)
  Top 0.152: v16.86,47.88 17.78,48.8 17.78,49.79 15.5,52.07 R17.2 | IC1.1 11.41,36.89 v11.49,36.89
  Bottom 0.152: v16.86,47.88 16.03,47.05 16.03,38.89 14.03,36.89 v11.49,36.89
AT_POCI
  Top 0.152: U3.20 12.7,52.85 12.7,53.34 J3.1
D+  (via drill 0.3)
  Top 0.224: IC1.2 9.78,36.79 v9.78,37.08 | v1.4,7.75 1.66,7.49 D3.1
  Bottom 0.224: v9.78,37.08 9.53,36.83 6.35,36.83 3.68,34.16 3.68,11.29 1.14,8.74 1.14,8 v1.4,7.75
D+_IN  (via drill 0.3)
  Top 0.224: J1.A6 11.18,7.12 v11.68,7.62 12.18,7.12 J1.B6 | D3.6 3.55,7.49 v3.68,7.62
  Bottom 0.224: v3.68,7.62 3.81,7.62 3.94,7.75 3.94,8.38 5.21,9.65 10.67,9.65 11.43,8.89 11.43,7.87 v11.68,7.62 11.68,7.59 11.43,7.34 11.43,6.63 11.81,6.25 11.81,3.94 11.94,3.81 D+.1
D-  (via drill 0.3)
  Top 0.224: IC1.3 9.02,36.85 v9.02,37.47 | v1.4,6.22 1.66,6.49 D3.3
  Bottom 0.224: v9.02,37.47 8.76,37.21 6.21,37.21 3.3,34.3 3.3,11.43 0.76,8.89 0.76,6.86 v1.4,6.22
D-_IN  (via drill 0.3)
  Top 0.224: D3.4 3.55,6.49 v3.68,6.35 | J1.B7 10.68,5.58 v11.18,5.08 11.68,5.58 J1.A7
  Bottom 0.224: v3.68,6.35 3.68,6.86 4.32,7.49 4.32,8.27 5.32,9.27 10.54,9.27 11.05,8.76 11.05,6.35 11.43,5.97 11.43,5.33 v11.18,5.08 11.43,4.83 11.43,3.94 11.3,3.81 D-.1
GND  (via drill 0.3)
  Top 0.152: U2.EPAD 4.83,26.92 U2.7 2.99,26.92 2.98,26.92 | IC1.28 15.15,33.91 15.56,33.91 v16.07,33.4 | U5.EPAD 9.91,26.92 U5.7 7.87,26.92 C11.2 | U4.7 16.26,26.92 U4.EPAD | v11.43,34.42 IC1.EPAD v10.03,33.02 | U2.6 3.39,27.77 2.98,27.37 2.98,26.92 | 2.98,26.92 2.98,25.02 3.3,24.7 v4.38,24.7 5.21,24.7 5.58,25.07 U2.12 | Q2.2 5,35.7 4.7,35.4 v4.7,34.04
  Top 0.203: U4.7 14.54,26.92 14.54,27.75 v14.61,27.81
  Top 0.254: C13.2 v7.62,50.8 | U3.PAD U3.8 9.78,48.51 v9.14,48.51 | D3.2 v1.4,6.99 | J2.10 17.21,23.69 v17.53,23.37 17.65,23.24 18.17,23.24 C8.2
  Top 0.305: C17.1 15.84,35.52 18,35.52 v18.03,35.56
  Bottom 0.152: v7.62,38.73 7.62,39.44 7.64,39.46 7.64,43.08 7.95,43.38 9.96,43.38 10.16,43.18 v10.16,41.78 | v4.45,31.75 4,31.3 4,25.09 v4.38,24.7
  other vias: 12.19,39.75 11.43,33.02 11.43,50.16 17.34,41.08 18.54,43.5 20.64,45.72 11.18,44.45 5.08,7.62 17.4,7.24 15.24,7.62 8.51,7.62 12.7,7.62 5.71,40.26 3.17,38.1 4.7,42.93 6.6,41.91 2.54,53.34 13.97,53.34 5.97,45.97 13.34,44.45 19.94,12.95 2.54,43.18 2.54,48.26 17.14,51.18 15.24,48.26 19.05,48.26 7.62,27.94 6.35,22.61 16.13,30.86 3.17,39.75 19.05,52.07 15.62,19.18 13.97,25.4 18.16,19.18 9.53,16.51 2.54,20.32 2.54,12.7 1.91,10.79 15.75,10.41 13.34,16.51 9.53,20.32 6.35,15.24 13.97,12.7 10.16,2.54 10.16,7.62 13.34,20.32 12.7,24.13 3.3,50.8 12.7,27.94 17.78,39.37 15.49,40.01 4.45,12.06 2.54,16.51 4.45,16.51 4.45,20.32 12.7,33.02 11.43,31.75 3.17,9.53 2.54,5.71 7.62,10.54 12.7,2.54 15.18,35.12 19.81,43.37
  pour Top (isolate 0.152, rank 3): 0,58.42 22.86,58.42 22.86,0 0,0
  pour Bottom (isolate 0.152, rank 2): 0,58.42 22.86,58.42 22.86,0 0,0
  pour Route2 (isolate 0.203, rank 2): 0,58.42 22.86,58.42 22.86,0 0,0
GPIO2  (via drill 0.3)
  Top 0.152: IC1.27 15.26,32.96 v15.26,33 | v11.3,41.78 R13.2
  Bottom 0.152: v15.26,33 13.99,33 10.67,36.32 10.67,41.15 v11.3,41.78 12.06,42.55 U6.5
GPIO4
  Top 0.152: IC1.29 14.82,34.29 16.64,34.29 R25.1
GPIO7  (via drill 0.3)
  Top 0.152: v11.3,40.77 R14.2 | IC1.31 13.73,34.68 v14.48,35.43
  Bottom 0.152: v14.48,35.43 14.22,35.18 12.28,35.18 10.95,36.5 10.95,40.41 v11.3,40.77 11.81,41.27 U6.6
GPIO10  (via drill 0.3)
  Top 0.152: IC1.21 13.16,29.87 v13.16,29.59
  Bottom 0.152: v13.16,29.59 13.16,30.02 12.7,30.48 GPIO10.1
MICROSD_CLK/SCK  (via drill 0.3)
  Top 0.152: U3.12 13.13,47.76 v13.13,47.3 | v2.31,22.48 3.43,22.48 5.84,24.89 9.16,24.89 | J2.5 v15.06,18.09 13.97,19.18 13.97,21.2 12.84,22.33 10.3,22.33 9.16,23.46 9.16,24.89 | 9.16,24.89 U5.9 | U4.10 16.01,24.9 v15.88,24.77
  Bottom 0.152: v2.31,22.48 2.56,22.73 2.56,34.82 5.87,38.13 5.91,38.13 7.36,39.58 7.36,43.29 7.74,43.66 11.66,43.66 12.32,44.32 12.32,46.49 v13.13,47.3 | v15.88,24.77 15.37,24.77 14.8,24.2 14.8,18.34 v15.06,18.09
MICROSD_CMD/SDI  (via drill 0.3)
  Top 0.152: U4.9 15.51,25.16 15.11,24.77 v14.48,24.77 13.72,24.77 13.34,25.15 13.34,28.07 12.45,28.96 10.92,28.96 10.66,28.69 U5.3 | J2.3 14.49,15.89 v14.48,15.88
  Bottom 0.152: v14.48,15.88 v14.48,24.77
MICROSD_D0/SDO
  Top 0.152: U4.2 17.51,28.3 17.65,28.45 18.92,28.45 19.68,27.69 19.68,20.95 19.02,20.29 J2.7 15.27,20.29 12.95,22.61 10.41,22.61 9.66,23.36 U5.10
MICROSD_D1  (via drill 0.3)
  Top 0.152: U5.2 11.16,28.3 11.33,28.48 v11.94,28.48 | v14,22.24 14.85,21.39 J2.8
  Bottom 0.152: v11.94,28.48 12.93,28.48 13.34,28.07 13.34,22.9 v14,22.24
MICROSD_D2  (via drill 0.3)
  Top 0.152: U2.3 v5.58,28.54 v5.59,28.55 | J2.1 15.52,13.69 v15.49,13.72
  Bottom 0.152: v5.59,28.55 5.05,28.02 5.05,18.29 8.93,14.41 14.8,14.41 v15.49,13.72
MICROSD_D3/!CS!  (via drill 0.3)
  Top 0.152: v6.35,28.55 6.08,28.28 U2.2 | v15.49,14.73 15.55,14.79 J2.2 18.47,14.79 v18.54,14.86 | U4.3 17.01,28.31 17.42,28.73 19.04,28.73 19.96,27.8 19.96,19.84 v18.54,18.41
  Bottom 0.152: v6.35,28.55 5.33,27.54 5.33,18.41 9.02,14.73 v15.49,14.73 | v18.54,18.41 v18.54,14.86
MICROSD_PWR_EN  (via drill 0.3)
  Top 0.152: U3.5 8.87,51.31 v8.64,51.31 | v19.05,30.48 19.94,31.37 19.94,39.94 19.38,40.5 16.65,40.5 v16.51,40.64 | R26.1 v18.29,6.22
  Bottom 0.152: v8.64,51.31 8.65,51.33 9.33,51.33 9.53,51.53 13.93,51.53 17.53,47.93 17.53,44.96 16.51,43.94 v16.51,40.64 | v19.05,30.48 20.07,30.48 20.38,30.16 20.38,13.27 21.59,12.06 21.59,7.62 20.19,6.22 v18.29,6.22
MICROSD_VCC  (via drill 0.3)
  Top 0.254: Q3.3 18.59,10.58 v18.33,10.83 18.33,11.21 C5.1 19.18,13.08 19.81,13.71 19.81,16.38 19.21,16.99 J2.4
  Bottom 0.254: v18.33,10.83 18.33,10.88 MICROSD_VCC.1
N$1
  Top 0.152: R11.2 6.74,3.81 8.89,3.81 10.18,5.1 J1.A5
N$2
  Top 0.152: R10.2 15.87,3.81 14.41,3.81 13.18,5.04 J1.B5
N$3
  Top 0.152: C3.1 6.85,32.26 7.99,31.11 8.82,31.11 IC1.13
N$4
  Top 0.152: IC1.34 13.11,36.11 13.11,37.11 11.47,38.74 C4.1
N$5
  Top 0.152: Q5.2 Q5.5 8.89,41.66 9.02,41.53 9.4,41.53 9.54,41.67 Q5.6 10.49,42.38 R21.2
N$6
  Top 0.152: R26.2 R9.1 20.18,8.2 Q3.1
N$7
  Top 0.152: Q2.1 4,36.07 R27.1 R20.2
N$8
  Top 0.152: Q2.3 6.15,36.24 5.47,35.57 R28.1
N$9
  Bottom 0.152: JP1.1 J4.19
N$10
  Bottom 0.152: JP2.1 J4.20
N$11
  Bottom 0.152: JP3.1 J4.21
N$12
  Route2 0.406: J1.SHLD1 J1.SHLD3 | J1.SHLD2 J1.SHLD4
  Bottom 0.406: J1.SHLD3 7.3,1.38 SH.1 15.56,1.38 J1.SHLD4
N$13
  Top 0.254: R22.2 7.94,43.68 Q5.3 8.24,44.93 Q4.1
N$14  (via drill 0.3)
  Top 0.152: R19.2 4.95,49.92 v4.95,50.29
  Bottom 0.152: I2C.3 5.26,49.99 v4.95,50.29
N$15
  Top 0.152: Q7.2 Q7.5 Q7.6 17.48,42.38 R23.2
N$16  (via drill 0.3)
  Top 0.152: R18.1 4.95,51.68 v4.95,51.31
  Bottom 0.152: I2C.1 3.63,49.99 v4.95,51.31
N$17
  Top 0.152: R7.1 8.57,40.19 Q1.1 8.57,38.54 8.13,38.1 7.37,38.1 6.86,37.59 6.86,36.2 6.47,35.81 R28.2
N$18
  Top 0.152: D2.A R17.1
N$19  (via drill 0.3)
  Top 0.152: D2.C v16.51,57.78
  Bottom 0.152: LED2.2 16.38,57.66 v16.51,57.78
N$20
  Top 0.152: IC1.30 14.43,34.61 15.94,34.61 16.38,35.05 17.26,35.05 R29.1
N$22
  Top 0.152: D1.A R8.1
N$23
  Top 0.152: IC1.35 12.7,36.41 12.7,37.12 11.68,38.14 10.29,38.14 10.16,38.27 R16.2
N$25
  Bottom 0.152: RXD.1 J4.14
N$26
  Bottom 0.152: TXD.1 J4.15
N$27  (via drill 0.3)
  Top 0.152: D1.C v6.35,57.78
  Bottom 0.152: v6.35,57.78 6.48,57.66 LED1.2
N$28
  Top 0.152: Q6.1 15.22,44.93 Q7.3 15.22,43.81 14.1,42.68 R24.2
PICO  (via drill 0.3)
  Top 0.152: v14.73,25.53 14.73,26.31 14.84,26.42 U4.8
  Bottom 0.152: J4.17 21.45,41.91 17.25,37.71 17.25,31.08 19.55,28.78 19.55,24.68 19.09,24.23 17.64,24.23 17.27,24.59 17.27,24.88 16.62,25.53 v14.73,25.53
POCI  (via drill 0.3)
  Top 0.152: U4.1 17.86,27.22 v18.41,27.77 | R30.2 21.2,44.45 J4.16
  Bottom 0.152: J4.16 20.19,43.05 20.19,41.05 16.97,37.82 16.97,30.93 18.41,29.49 v18.41,27.77
RXD0  (via drill 0.3)
  Top 0.152: U3.3 9.62,51.98 v9.62,52.29
  Bottom 0.152: v9.62,52.29 9.77,52.29 9.86,52.2 14.22,52.2 16.89,49.53 RXD.2
SCL
  Top 0.152: R19.1 J4.2 | U3.1 11.43,52.85 J3.3
  Bottom 0.152: J4.2 2.54,50.8 2.54,52.26 3.14,52.86 8.93,52.86 10.68,54.61 J3.3
SCLK  (via drill 0.3)
  Top 0.152: v16.56,24.77 16.51,24.81 U4.11
  Bottom 0.152: J4.18 19.3,39.37 17.53,37.59 17.53,31.2 19.82,28.9 19.82,24.57 19.22,23.96 19.21,23.95 17.37,23.95 v16.56,24.77
SD_!CD!  (via drill 0.3)
  Top 0.152: J2.9 16.84,22.48 v15.49,22.48 | IC1.26 15.01,31.56 16.32,31.56 17.08,30.8 17.08,29.32 17.4,29.01 19.04,29.01 v19.75,29.72
  Bottom 0.152: v19.75,29.72 20.1,29.36 20.1,23.79 18.8,22.48 v15.49,22.48
SD_CLK  (via drill 0.3)
  Top 0.152: IC1.9 7.69,33.17 4.58,33.17 3.68,32.27 3.68,29.7 4.19,29.19 v4.54,29.19 | v8.38,25.65 8.38,26.12 8.68,26.42 U5.8
  Bottom 0.152: v4.54,29.19 4.94,29.59 6.6,29.59 7.14,29.06 7.14,26.64 8.13,25.65 v8.38,25.65
SD_CMD
  Top 0.152: IC1.11 8.04,31.75 7.87,31.75 6.73,32.89 4.7,32.89 3.96,32.16 3.96,30.45 4.83,29.59 9.61,29.59 10.16,29.04 U5.4
SD_D0  (via drill 0.3)
  Top 0.152: IC1.5 9.02,35.43 8.13,35.43 v7.75,35.81 | v10.16,24.77 U5.11
  Bottom 0.152: v7.75,35.81 7.75,35.79 7.14,35.18 7.14,30.07 7.89,29.32 7.89,28.49 8.33,28.05 8.59,28.05 9.21,27.43 9.21,25.08 9.53,24.77 v10.16,24.77
SD_D1  (via drill 0.3)
  Top 0.152: IC1.4 9.23,35.93 v8.62,35.93 | v11.94,27.69 11.94,27.09 11.76,26.92 U5.1
  Bottom 0.152: v11.94,27.69 11.3,28.33 8.45,28.33 8.17,28.61 8.17,29.88 7.49,30.55 7.49,35.04 7.76,35.31 8.51,35.31 8.62,35.42 v8.62,35.93
SD_D2  (via drill 0.3)
  Top 0.152: U2.4 5.08,28.78 5.59,29.29 9.25,29.29 9.33,29.21 v9.33,29.09 | v15.3,30.86 14.99,30.86 14.08,31.77 IC1.25
  Bottom 0.152: v15.3,30.86 15.05,31.11 14.35,31.11 13.97,30.73 13.97,30.23 14.35,29.84 14.35,29.21 14.18,29.04 12.45,29.04 12.18,29.31 10.06,29.31 9.84,29.09 v9.33,29.09
SD_D3  (via drill 0.3)
  Top 0.152: IC1.23 | v14.48,30.48 13.97,30.48 IC1.23 | v8.65,28.81 7.47,28.81 6.86,28.19 6.86,27.09 6.68,26.92 U2.1
  Bottom 0.152: v8.65,28.81 8.85,28.61 9.75,28.61 10.18,29.03 12.06,29.03 12.34,28.75 14.4,28.75 14.73,29.08 14.73,30.23 v14.48,30.48
SDA  (via drill 0.3)
  Top 0.152: J4.1 R18.2 4.83,53.34 v5.08,53.34 | J3.4 12.7,55.88 13.97,55.88 14.73,55.12 14.73,52.05 U3.16
  Bottom 0.152: v5.08,53.34 9.02,53.34 10.16,54.48 10.16,55.88 J3.4
SDIO_!RESET!  (via drill 0.3)
  Top 0.152: IC1.18 10.57,29.34 10.29,29.34 9.53,30.1 v8.76,30.1 6.36,30.1 R1.2 C16.1
  Bottom 0.152: v8.76,30.1 9.27,30.1 9.65,30.48 SDIO_!RESET!.1
SDIO_EN  (via drill 0.3)
  Top 0.152: U3.2 10.18,52.12 v10.18,52.81 | U2.5 v4.58,28.5 v4.57,28.51 4,28.51 3.25,29.26 3.25,36.39 R27.2 4.43,37.57 5.57,37.57 5.71,37.72 v5.71,38.61 | U5.12 10.66,25.03 v10.92,24.77 11.16,25 U5.13 | v8.38,27.57 8.59,27.77 U5.6 9.16,28.34 9.27,28.45 9.53,28.45 9.66,28.31 U5.5 | U2.13 6.77,25.57 v6.86,25.65
  Bottom 0.152: v10.18,52.81 9.29,52.81 8.98,52.5 7.18,52.5 6.63,51.95 6.63,43.46 5.08,41.91 5.08,39.37 5.71,38.73 v5.71,38.61 | v4.57,28.51 4.76,28.51 5.41,29.16 6.53,29.16 6.86,28.83 v6.86,25.65 6.86,25.27 7.85,24.29 8.89,24.29 | v10.92,24.77 10.44,24.29 8.89,24.29 | v8.38,27.57 8.89,27.06 8.89,24.29
SDIO_VDD  (via drill 0.3)
  Top 0.152: IC1.6 8.69,35.05 8.26,35.05 v8,34.8 | IC1.22 13.84,29.9 v13.84,29.59 14.99,29.59 C14.1 | IC1.36 12.19,36.61 12.19,37.21 11.81,37.59 v11.43,37.59 9.91,37.59 9.53,37.97 8.59,37.97 Q1.3 7.62,36.43 7.2,36.01 7.2,35.41 7.81,34.8 v8,34.8 | R1.1 6.87,31.23 7.46,30.64 v8.1,30.64 9.04,30.64 IC1.14 | R13.1 13.07,41.55 R14.1 13.09,40.75 C19.1 v13.08,38.73 | C15.1 7.24,34.04 v8,34.8
  Bottom 0.152: v13.84,29.59 13.84,29.84 13.46,30.23 13.46,30.99 13.34,31.11 10.79,31.11 SDIO_VDD.1 9.04,30.64 v8.1,30.64 7.85,30.89 7.85,34.64 v8,34.8 | U6.8 v13.08,38.73 11.94,37.59 v11.43,37.59
SPI_EN  (via drill 0.3)
  Top 0.152: U3.11 12.57,47.61 12.57,44.45 13.34,43.69 13.34,42.04 14.58,40.8 15.59,40.8 16.23,40.16 19.26,40.16 19.6,39.83 19.6,32.11 17.59,30.1 v17.59,29.59 | R15.2 13.97,27.94 14.61,28.57 v15.75,28.57 | U4.5 16.01,28.31 v15.75,28.57 | U4.13 17.51,25.16 v17.91,24.77 17.4,24.77 17.01,25.15 U4.12 | U4.6 15.51,28.34 v15.75,28.57
  Bottom 0.152: v15.75,28.57 15.75,27.88 | 15.75,27.88 15.75,26.92 v17.91,24.77 | v17.59,29.59 17.59,28.7 16.76,27.88 15.75,27.88
TXD0  (via drill 0.3)
  Top 0.152: U3.4 9.13,51.75 v9.13,51.8
  Bottom 0.152: v9.13,51.8 14.11,51.8 18.64,47.27 TXD.2
V_USB  (via drill 0.3)
  Top 0.254: 2.54,39.24 2.54,40.67 U1.1 3.75,43.12 4.19,43.56 5.21,43.56 5.65,43.12 U1.3 | 4.32,9.78 1.78,12.32 1.78,22.73 2.54,23.5 2.54,39.24 | 4.32,9.78 9.14,9.78 | 9.14,9.78 13.08,9.78 13.88,8.98 v13.88,7.62 J1.VBUS2 | 9.14,9.78 9.14,6.49 J1.VBUS1 | 2.54,39.24 2.6,39.18 R2.2 C6.1 | 4.32,9.78 4.32,7.24 4.06,6.99 D3.5
  Bottom 0.254: V_USB.1 14.35,3.81 13.34,4.83 13.34,7.08 v13.88,7.62
V_USB_DIV_2  (via drill 0.3)
  Top 0.152: R3.2 R2.1 5.26,39.5 v5.71,39.5 | U3.14 13.53,48.77 v13.97,48.77
  Bottom 0.152: v13.97,48.77 13.97,48.22 13.53,47.78 12.88,47.78 11.97,46.86 11.97,44.49 11.42,43.94 7.62,43.94 7.08,43.41 7.08,40.61 5.97,39.5 v5.71,39.5
VCC  (via drill 0.3)
  Top 0.152: R9.2 19.18,8.39 19.68,8.89 v19.68,10.67
  Top 0.254: Q1.2 6.67,40.19 R7.2 | Q5.4 8.24,42.25 7.12,41.13 R7.2 | v9.78,46.23 9.84,46.17 Q4.2 | C18.1 16.83,45.22 Q6.2 16.82,46.1 v16.76,46.16 | v15.49,41.4 15.22,41.67 Q7.4 | U2.14 7.37,26.42 C11.1 v7.62,25.4 | v12.7,25.4 C9.1 12.45,26.42 U5.14 | Q3.2 20.62,10.67 v19.68,10.67 | R7.2 v6.35,40.64 | v7.62,48.26 C13.1 R4.2 6.47,49.03 5.71,49.78 5.71,50.73 v5.79,50.8 7.36,52.37 R8.2 | U3.9 9.85,47.88 v9.78,47.88 | U4.14 18.28,26.42 18.41,26.29 v18.41,25.46 18.67,25.21 18.67,24.26 C8.1
  Bottom 0.152: I2C.2 v4.45,48.26
  pour Route15 (isolate 0.203): 0,0 0,58.42 22.86,58.42 22.86,0
VCC_1
  Top 0.254: U1.5 3.75,45.78 C7.1 3.94,45.98 3.94,46.48 4.78,47.33 Q4.3 | Q4.3 10.32,47.33 C1.1 | Q5.1 9.54,44.31 8.89,44.96 Q4.3
XTAL1
  Top 0.152: IC1.33 13.02,35.38 14.38,36.74 R12.2 14.38,38.4 C12.2 14.9,39.03 Y1.3
XTAL2
  Top 0.152: IC1.32 13.38,35.03 14.7,36.35 R12.1 16.43,36.35 C17.2 16.48,36.68 16.76,36.95 Y1.1

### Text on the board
Top: 1
Route2: 2
Route15: 3
Bottom: v10 | 4
Measures: Dimensions in Inches
tDocu: 4-Layer Board / 1.6mm Thickness / 1oz Copper (Outer layers) / LeadFree HASL Finish | Paul Clark

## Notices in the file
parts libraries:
SparkFun-Aesthetics: Licensing: Creative Commons ShareAlike 4.0 International - https://creativecommons.org/licenses/by-sa/4.0
SparkFun-Aesthetics: Released under the Creative Commons Attribution Share-Alike 4.0 License
SparkFun-Aesthetics: https://creativecommons.org/licenses/by-sa/4.0
